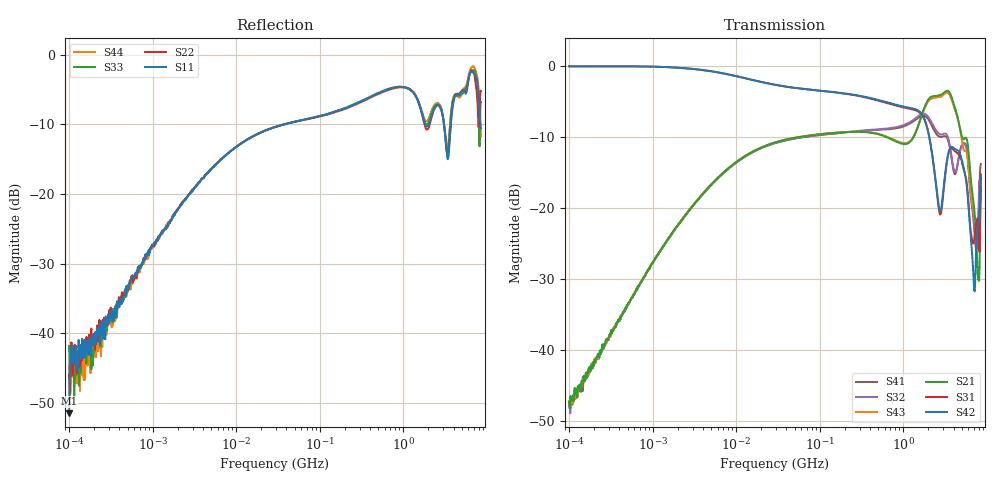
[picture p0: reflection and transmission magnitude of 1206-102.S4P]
!Agilent Technologies,E5071C,MY46110495,A.10.06
!Date: Tue Jun 06 11:15:25 2017
!Data & Calibration Information:
!Freq	S11:SOLT4(ON)	S12:SOLT4(ON)	S13:SOLT4(ON)	S14:SOLT4(ON)
!	S21:SOLT4(ON)	S22:SOLT4(ON)	S23:SOLT4(ON)	S24:SOLT4(ON)
!	S31:SOLT4(ON)	S32:SOLT4(ON)	S33:SOLT4(ON)	S34:SOLT4(ON)
!	S41:SOLT4(ON)	S42:SOLT4(ON)	S43:SOLT4(ON)	S44:SOLT4(ON)
!PortZ  Port1:50+j0  Port2:50+j0  Port3:50+j0  Port4:50+j0
!Above PortZ is port z conversion or system Z0 setting when saving the data.
!When reading, reference impedance value at option line is always used.
# Hz S dB R 50
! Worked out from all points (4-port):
!   801 points, 100 kHz to 8.5 GHz, reference 50 ohm
!   strongest paths, dB at 100 kHz, 1.721 MHz, 29.51 MHz, 502.3 MHz, 8.5 GHz:
!     S42: 0.0, -0.2, -2.7, -4.8, -15.6
!     S31: -0.1, -0.2, -2.7, -4.9, -15.3
!     S21: -47.4, -23.5, -10.8, -9.6, -17.5
!     S43: -47.2, -23.5, -10.8, -9.6, -16.3
!     S32: -47.9, -23.6, -10.9, -8.9, -17.1
!     S41: -47.9, -23.6, -10.9, -9.0, -13.9
!   lowest |S11| = -51.5 dB at 100 kHz (marker M1), VSWR 1.01, Z = 50.1 + j0.237 ohm
!   |S11| at or under -10 dB: start of sweep to 38.49 MHz; 1.832 GHz to 2.026 GHz (193.1 MHz wide, 10 % of centre); 3.068 GHz to 3.711 GHz (642.3 MHz wide, 18.9 % of centre)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
100000  -51.50 62.9  -47.57 85.2  -0.05 -0.1  -47.50 -96.1
        -47.37 90.3  -46.01 39.6  -48.19 -89.6  -0.07 -0.0
        -0.07 -0.1  -47.92 -92.9  -41.86 91.9  -47.66 88.6
        -47.92 -90.8  -0.04 -0.1  -47.24 84.8  -44.79 78.5
1.799738e7  -11.41 31.6  -11.76 29.1  -2.14 -10.3  -11.83 -151.9
            -11.75 29.1  -11.40 31.2  -11.84 -151.9  -2.15 -10.2
            -2.15 -10.3  -11.85 -151.8  -11.42 31.6  -11.75 29.0
            -11.82 -151.9  -2.15 -10.2  -11.74 29.0  -11.41 31.2
1.083427e9  -4.80 31.2  -11.01 15.5  -5.94 -39.9  -8.40 129.0
            -11.01 15.5  -4.73 30.7  -8.19 128.8  -5.83 -39.0
            -5.94 -39.8  -8.21 128.8  -4.75 29.2  -10.90 12.6
            -8.39 129.1  -5.81 -39.0  -10.88 12.7  -4.81 31.8
2.570722e9  -7.22 99.2  -4.22 4.3  -18.65 -88.0  -9.79 49.5
            -4.22 4.4  -7.27 100.6  -9.35 47.0  -18.39 -84.2
            -18.70 -88.0  -9.35 47.1  -7.15 96.0  -4.44 -0.6
            -9.80 49.6  -18.38 -84.3  -4.43 -0.7  -6.93 96.6
5.086878e9  -5.21 -85.6  -10.09 -47.9  -13.71 -149.5  -11.12 3.3
            -10.09 -47.9  -5.11 -85.2  -11.13 -1.4  -13.52 -144.6
            -13.74 -149.4  -11.14 -1.3  -5.67 -82.9  -10.87 -64.9
            -11.12 3.6  -13.51 -144.5  -10.87 -64.7  -5.31 -77.0
6.738951e9  -2.51 8.6  -18.10 -78.0  -24.73 84.7  -20.37 -49.0
            -18.07 -78.0  -2.31 4.5  -19.73 -51.6  -27.23 80.4
            -24.77 85.0  -19.72 -51.4  -2.34 7.1  -19.70 -81.1
            -20.34 -48.6  -27.20 80.9  -19.67 -81.0  -1.73 9.5
8.5e9  -10.60 107.7  -17.48 120.3  -15.29 89.9  -13.84 -15.4
       -17.52 120.4  -5.31 111.4  -17.09 -11.5  -15.59 95.8
       -15.29 90.1  -17.09 -11.3  -6.83 126.6  -16.34 133.7
       -13.86 -15.0  -15.58 96.2  -16.34 133.8  -11.75 88.6
